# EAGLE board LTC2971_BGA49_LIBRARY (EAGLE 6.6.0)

No outline drawn. Coordinates in mm, seen from the top.
Copper layers (1*2+15*16): Top 0.06mm / dielectric 0.2mm / Route2 0.035mm / dielectric 0.15mm / Route15 0.035mm / dielectric 0.2mm / Bottom 0.06mm
Design rules "default": minimum track width 10mil, minimum drill 24mil, track to track 8mil, track to pad 8mil, pad to pad 8mil, via to via 8mil, smd to smd 8mil, copper to edge 40mil, drill to drill 8mil, minimum pad ring 10mil, minimum via ring 8mil, stop-mask expansion 4mil, vias tented up to drill 0mil, thermal gap 10mil

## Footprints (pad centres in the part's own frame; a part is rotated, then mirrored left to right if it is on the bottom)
BGA49 = smd 0.47 x 0.47: A1 -3,3; A2 -2,3; A3 -1,3; A4 0,3; A5 1,3; A6 2,3; A7 3,3; B1 -3,2; B2 -2,2; B3 -1,2; B4 0,2; B5 1,2; B6 2,2; B7 3,2; C1 -3,1; C2 -2,1; C3 -1,1; C4 0,1; C5 1,1; C6 2,1; C7 3,1; D1 -3,0; D2 -2,0; D3 -1,0; D4 0,0; D5 1,0; D6 2,0; D7 3,0; E1 -3,-1; E2 -2,-1; E3 -1,-1; E4 0,-1; E5 1,-1; E6 2,-1; E7 3,-1; F1 -3,-2; F2 -2,-2; F3 -1,-2; F4 0,-2; F5 1,-2; F6 2,-2; F7 3,-2; G1 -3,-3; G2 -2,-3; G3 -1,-3; G4 0,-3; G5 1,-3; G6 2,-3; G7 3,-3

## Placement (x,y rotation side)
U1  [BGA49]  4,4 0 top

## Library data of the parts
U1 = linear-technology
